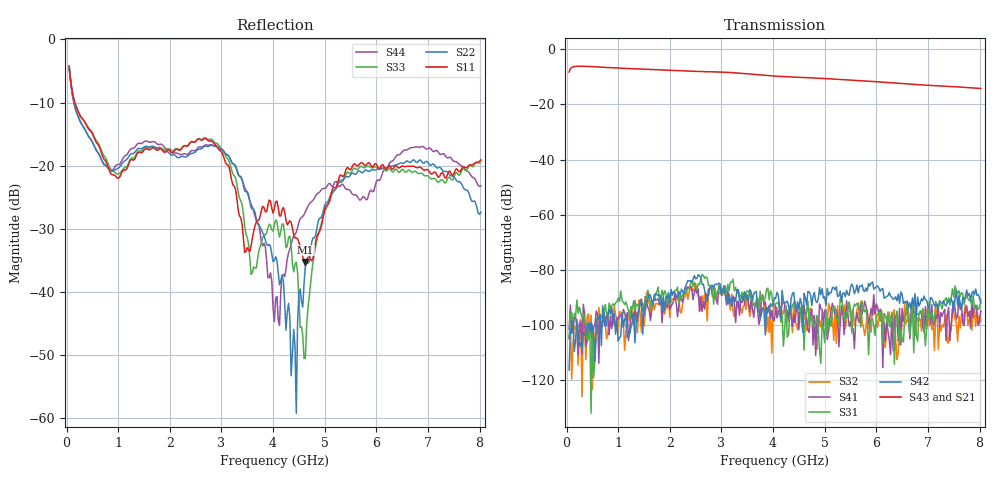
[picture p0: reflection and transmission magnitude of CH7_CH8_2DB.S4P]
!Agilent Technologies,E5071C,MY46316741,A.11.02
!Date: Mon Jun 01 10:29:37 2026
!Data & Calibration Information:
!1:CH7 INPUT 2:CH7 OUTPUT 3:CH8 INPUT 4:CH8 OUTPUT
!Freq	S11:SOLT4(ON)	S12:SOLT4(ON)	S13:SOLT4(ON)	S14:SOLT4(ON)
!	S21:SOLT4(ON)	S22:SOLT4(ON)	S23:SOLT4(ON)	S24:SOLT4(ON)
!	S31:SOLT4(ON)	S32:SOLT4(ON)	S33:SOLT4(ON)	S34:SOLT4(ON)
!	S41:SOLT4(ON)	S42:SOLT4(ON)	S43:SOLT4(ON)	S44:SOLT4(ON)
!PortZ  Port1:50+j0  Port2:50+j0  Port3:50+j0  Port4:50+j0
!Above PortZ is port z conversion or system Z0 setting when saving the data.
!When reading, reference impedance value at option line is always used.
# Hz S dB R 50
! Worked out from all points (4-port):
!   320 points, 50 MHz to 8.025 GHz, reference 50 ohm
!   strongest paths, dB at 50 MHz, 2.05 GHz, 4.05 GHz, 6.05 GHz, 8.025 GHz:
!     S43: -8.3, -7.7, -9.8, -11.9, -14.3
!     S21: -8.3, -7.8, -9.9, -12.1, -14.4
!     S42: -116.4, -89.2, -90.4, -86.6, -92.0
!     S31: -105.0, -88.5, -92.4, -95.3, -90.7
!     S41: -101.4, -92.5, -93.2, -95.9, -94.8
!     S32: -104.8, -90.6, -94.5, -97.4, -98.5
!   lowest |S11| = -35.3 dB at 4.625 GHz (marker M1), VSWR 1.03, Z = 51.4 + j1.07 ohm
!   |S11| at or under -10 dB: 159.3 MHz to end of sweep
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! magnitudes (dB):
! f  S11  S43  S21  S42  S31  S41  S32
! 50 MHz  -4.2  -8.3  -8.3  -116.4  -105.0  -101.4  -104.8
! 3.25 GHz  -23.3  -8.6  -8.7  -90.0  -87.6  -91.6  -97.1
! 4.025 GHz  -26.8  -9.8  -9.9  -90.1  -92.9  -98.5  -92.1
! 4.45 GHz  -31.5  -10.2  -10.3  -95.1  -95.0  -94.1  -99.4
! 4.625 GHz  -35.3  -10.3  -10.4  -90.2  -97.9  -95.9  -96.5
! 5.425 GHz  -20.4  -11.1  -11.3  -87.4  -95.9  -91.2  -97.3
! 8.025 GHz  -19.1  -14.3  -14.4  -92.0  -90.7  -94.8  -98.5
